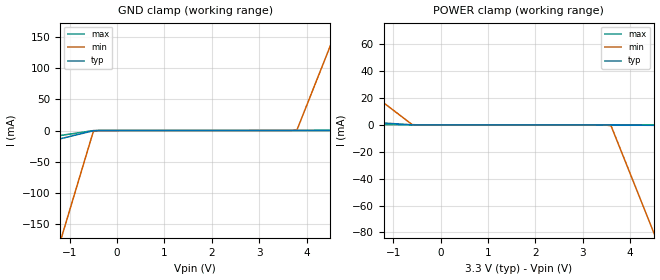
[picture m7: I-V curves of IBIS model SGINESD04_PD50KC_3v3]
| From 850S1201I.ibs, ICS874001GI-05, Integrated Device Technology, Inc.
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[Model] SGINESD04_PD50KC_3v3
Model_type   Input
Polarity   Non-Inverting
Vinl = 0.80V
Vinh = 2.2V
|   typ   min   max
C_comp   2pF   1.5pF   2.5pF
|   typ   min   max
[Voltage range]  3.3V   3.135V   3.465V
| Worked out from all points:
|   GND clamp passes 1 mA (typ) near -0.53 V on its own axis
|   POWER clamp passes 1 mA (typ) near -0.99 V on its own axis
[GND_clamp]
|Voltage   I(typ)   I(min)   I(max)
-3.3V     -52.25mA   -711.5mA   -31.55mA
-1.2V     -13.34mA   -179.1mA   -8.006mA
-1.1V     -11.49mA   -153.7mA   -6.884mA
-500mV    -368.1uA   -1.645mA   -156.4uA
-300mV    -6.904uA   -14.83uA   -5.752uA
3.6V      71.67uA    84.28uA    68.21uA
3.8V      77.35uA    1.187mA    72.01uA
4.6V      279.8uA    154.8mA    87.25uA
4.7V      305.1uA    174mA      89.15uA
6.6V      785.9uA    539mA      125.3uA
[POWER_clamp]
|Voltage   I(typ)   I(min)   I(max)
-3.3V     6.274mA    73.01mA    1.235mA
-600mV    102.7uA    302.6uA    79.58uA
3.4V      -1.989uA   -8.579uA   1.23uA
3.6V      -6.904uA   -691.8uA   -2.555uA
4.5V      -247.9uA   -80.18mA   -19.62uA
4.6V      -274.7uA   -89.02mA   -21.52uA
6.6V      -810.3uA   -265.7mA   -59.45uA
